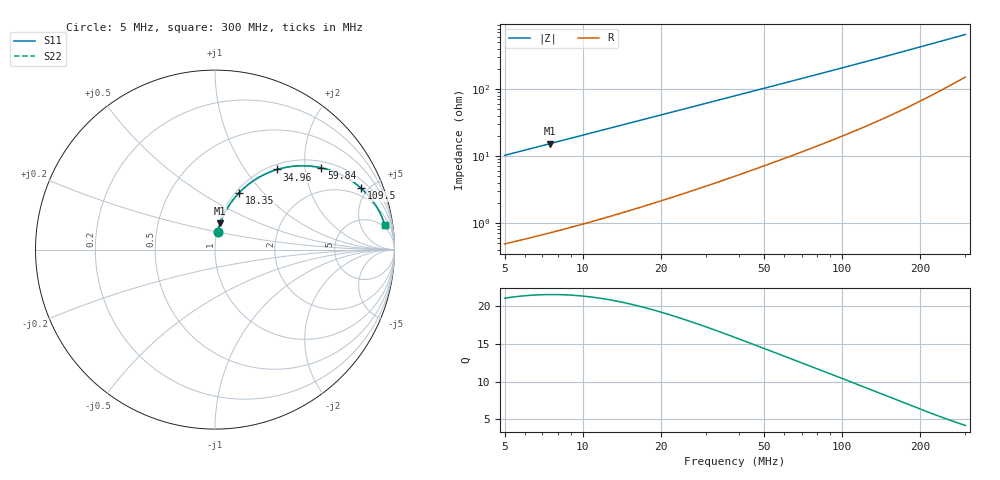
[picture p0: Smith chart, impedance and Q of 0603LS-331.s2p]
# MHz S MA R 50
!Freq  MagS11  AngS11  MagS21  AngS21  MagS12  AngS12  MagS22  AngS22
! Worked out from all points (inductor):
!   801 points, 5 MHz to 300 MHz, reference 50 ohm
!   read as one part in series: L = 325 nH near 5.103 MHz
!   highest Q = 21.5 at 7.453 MHz (marker M1), where L = 325 nH
!   S11 on the Smith chart (normalised r, x): 5 MHz: 1.01, +0.20; 18.35 MHz: 1.04, +0.75; 34.96 MHz: 1.09, +1.43; 59.84 MHz: 1.18, +2.44; 109.5 MHz: 1.45, +4.50; 300 MHz: 4, +13
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5  0.1011 81.5  0.9901 -5.8  0.9901 -5.8  0.1011 81.5
6.230826  0.1254 80.1  0.9863 -7.2  0.9863 -7.2  0.1254 80.1
7.453148  0.1494 78.8  0.9819 -8.6  0.9819 -8.6  0.1494 78.8
9.626628  0.1911 76.3  0.9727 -11.0  0.9727 -11.0  0.1911 76.3
12.11979  0.2375 73.5  0.9601 -13.7  0.9601 -13.7  0.2375 73.5
15.02616  0.2892 70.4  0.9431 -16.8  0.9431 -16.8  0.2892 70.4
18.34565  0.3449 66.9  0.9212 -20.1  0.9212 -20.1  0.3449 66.9
21.83255  0.3992 63.5  0.8959 -23.5  0.8959 -23.5  0.3992 63.5
25.7176  0.4546 59.8  0.8659 -27.0  0.8659 -27.0  0.4546 59.8
34.96164  0.5651 52.2  0.7914 -34.3  0.7914 -34.3  0.5651 52.2
43.79153  0.6461 46.1  0.7219 -40.1  0.7219 -40.1  0.6461 46.1
54.29291  0.7181 40.1  0.6464 -45.7  0.6464 -45.7  0.7181 40.1
59.8376  0.7479 37.5  0.6104 -48.2  0.6104 -48.2  0.7479 37.5
69.41162  0.7892 33.6  0.5545 -51.9  0.5545 -51.9  0.7892 33.6
79.69752  0.8229 30.1  0.5027 -55.1  0.5027 -55.1  0.8229 30.1
103.467  0.8736 24.0  0.409 -60.4  0.409 -60.4  0.8736 24.0
109.459  0.8825 22.8  0.39 -61.4  0.39 -61.4  0.8825 22.8
128.937  0.9046 19.6  0.3377 -64.0  0.3377 -64.0  0.9046 19.6
152.6604  0.9222 16.7  0.2888 -66.2  0.2888 -66.2  0.9222 16.7
202.2899  0.9421 12.5  0.2193 -68.5  0.2193 -68.5  0.9421 12.5
252.0866  0.9514 9.9  0.1752 -69.0  0.1752 -69.0  0.9514 9.9
300  0.9561 8.2  0.1462 -68.5  0.1462 -68.5  0.9561 8.2
